(* Logix 5000 AddOnInstructionDefinition export AMCI_MAS; software revision 20.05 *)

TYPE AMCI_Motion_Axis_Output_Data :
STRUCT
   Control_Word_0 : INT;
   Control_Word_1 : INT;
   Position_or_Distance : DINT;
   Programmed_Speed : DINT;
   Acceleration : INT;
   Deceleration : INT;
   Output_Word_8 : INT;
   Output_Word_9 : INT;
END_STRUCT
END_TYPE

TYPE AMCI_Motion_Axis_Input_Data :
STRUCT
   Moving_CW : BOOL;
   Moving_CCW : BOOL;
   In_Hold_State : BOOL;
   Stopped : BOOL;
   At_Home : BOOL;
   Accelerating : BOOL;
   Decelerating : BOOL;
   Move_Complete : BOOL;
   Status_Word_0_Bit_8 : BOOL;
   Status_Word_0_Bit_9 : BOOL;
   Position_Invalid : BOOL;
   Input_Error : BOOL;
   Command_Error : BOOL;
   Configuration_Error : BOOL;
   Module_OK : BOOL;
   Mode_Flag : BOOL;
   IN1_Active : BOOL;
   IN2_Active : BOOL;
   IN3_Active : BOOL;
   IN4_Active : BOOL;
   Status_Word_1_Bit_4 : BOOL;
   Status_Word_1_Bit_5 : BOOL;
   Connection_Was_Lost : BOOL;
   Driver_Fault : BOOL;
   Status_Word_1_Bit_8 : BOOL;
   Invalid_Jog_Change : BOOL;
   Status_Word_1_Bit_10 : BOOL;
   Heartbeat_Bit : BOOL;
   Status_Word_1_Bit_12 : BOOL;
   Status_Word_1_Bit_13 : BOOL;
   Stall_Detected : BOOL;
   Drive_Is_Enabled : BOOL;
   Motor_Position : DINT;
   Encoder_Position : DINT;
   Trapped_Encoder_Position : DINT;
   Input_Word_8 : INT;
   Input_Word_9 : INT;
END_STRUCT
END_TYPE

ADD_ON_INSTRUCTION AMCI_MAS   (* revision 2.0, vendor AMCI, ExecuteEnableInFalse *)
// AMCI Motion Axis Stop
// Revision note:
// 3/12/2024 Version 2: Logic added to keep the driver in its current state, either enabled or disabled.
// Help:
// MOTION AXIS STOP: Stops motion that is occurring.
// AXIS INPUT DATA:  Input data from AMCI motion device.   Uses the AMCI_Motion_Axis_Input_Data User Defined Data Type.
// AXIS OUTPUT DATA; Output data from the AOI to the AMCI motion device.   Uses the AMCI_Motion_Axis_Output_Data User Defined Data Type.
// EN (Enable) Set when rung is true, Reset when rung is false
// DN (Done) Set when command is sent to the motion device.  Reset when the rung is false.
// ER (Error) Set when a command or input error failed to clear.  Reset when the rung is false.
// IP (In Process) Set when axis is decelerating.   Reset when motion stops or the rung goes false.
// PC (Process Complete) Set when motion has stopped.   Reset the next time the rung with the AOI transitions                                      from false to true.
VAR_IN_OUT
   Axis_Input_Data : AMCI_Motion_Axis_Input_Data; {required}
        [0].0   // set when moving CW
        [0].6   // set when axis is decelerating
        [1].0   // set when moving CCW
   Axis_Output_Data : AMCI_Motion_Axis_Output_Data; {required}
END_VAR
VAR_OUTPUT
   EN : BOOL; {visible}   // set when rung with AOI is true
   DN : BOOL; {access Read Only, visible}   // set when hold was succesfully initiated
   ER : BOOL; {visible}
   IP : BOOL; {visible}   // set when decelerating
   PC : BOOL; {visible}   // set when process complete
END_VAR
VAR
   command_data_block : INT[10];
        [0]   // Command Bits MSW
        [1]   // Command Bits LSW
        [2]   // Upper Target Position
        [3]   // Lower Target Position
        [4]   // Upper Programmed Speed
        [5]   // Lower Programmed Speed
   internal_enable : BOOL; {access None}   // set when driver ready to receive command
END_VAR

ROUTINE EnableInFalse   (* ladder *)
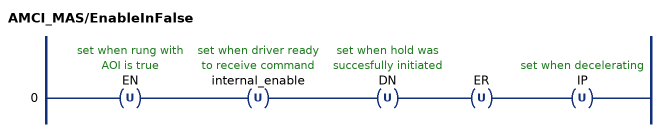
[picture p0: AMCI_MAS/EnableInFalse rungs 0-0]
   0: OTU(EN)OTU(internal_enable)OTU(DN)OTU(ER)OTU(IP);
END_ROUTINE

ROUTINE Logic   (* ladder *)
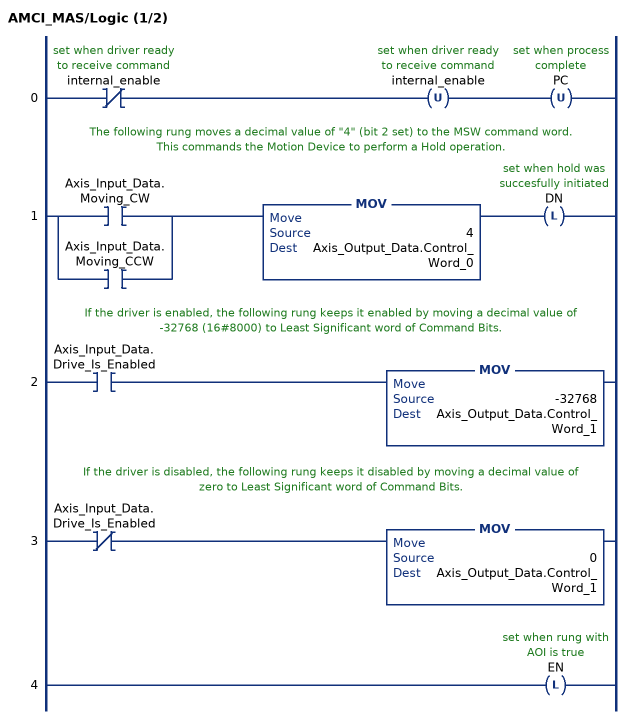
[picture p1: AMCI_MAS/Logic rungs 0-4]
   0: XIO(internal_enable)OTU(internal_enable)OTU(PC);
   // The following rung moves a decimal value of "4" (bit 2 set) to the MSW command word.  This commands the Motion Device to perform a Hold operation.
   1: [XIC(Axis_Input_Data.Moving_CW) ,XIC(Axis_Input_Data.Moving_CCW) ]MOV(4,Axis_Output_Data.Control_Word_0)OTL(DN);
   // If the driver is enabled, the following rung keeps it enabled by moving a decimal value of -32768 (16#8000) to Least Significant word of Command Bits.
   2: XIC(Axis_Input_Data.Drive_Is_Enabled)MOV(-32768,Axis_Output_Data.Control_Word_1);
   // If the driver is disabled, the following rung keeps it disabled by moving a decimal value of zero to Least Significant word of Command Bits.
   3: XIO(Axis_Input_Data.Drive_Is_Enabled)MOV(0,Axis_Output_Data.Control_Word_1);
   4: OTL(EN);
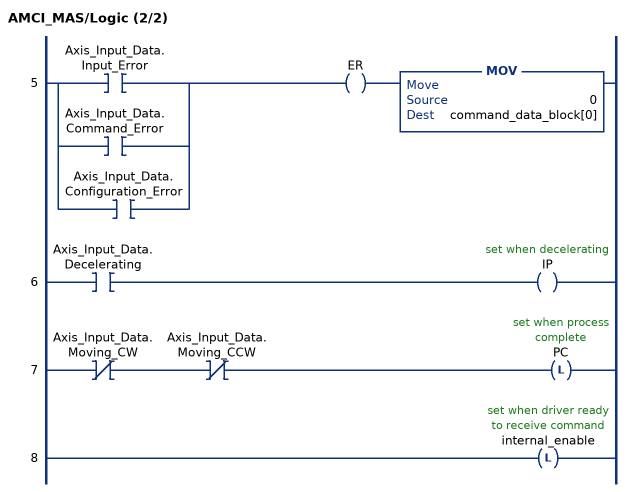
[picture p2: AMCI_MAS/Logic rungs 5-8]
   5: [XIC(Axis_Input_Data.Input_Error) ,XIC(Axis_Input_Data.Command_Error) ,XIC(Axis_Input_Data.Configuration_Error) ]OTE(ER)MOV(0,command_data_block[0]);
   6: XIC(Axis_Input_Data.Decelerating)OTE(IP);
   7: XIO(Axis_Input_Data.Moving_CW)XIO(Axis_Input_Data.Moving_CCW)OTL(PC);
   8: OTL(internal_enable);
END_ROUTINE
END_ADD_ON_INSTRUCTION
